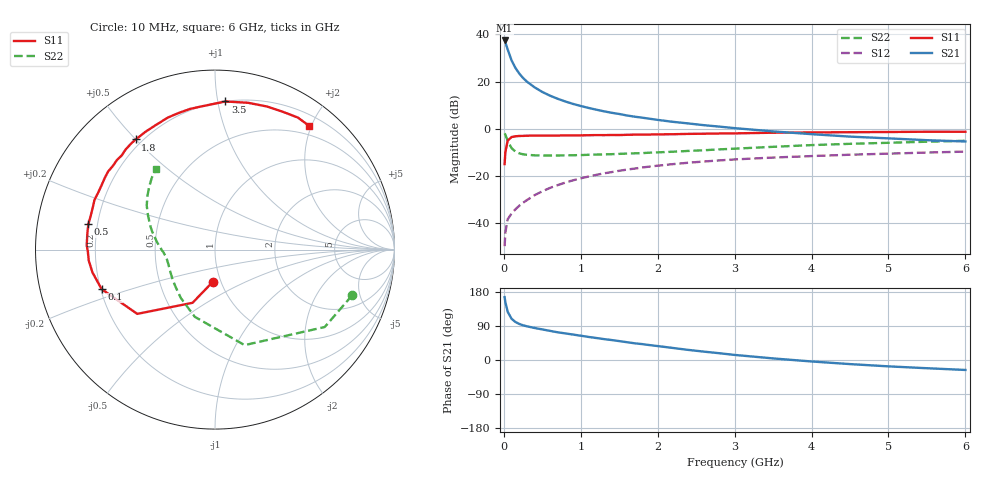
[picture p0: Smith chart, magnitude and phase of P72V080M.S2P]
! SIEMENS Small Signal Semiconductors
! BFP196
! Si NPN RF Bipolar Junction Transistor in SOT143
! VCE = 2 V  IC = 80 mA
! Common Emitter S-Parameters:  May  1996
# GHz  S  MA  R  50
!  f  S11  S21  S12  S22
! GHz  MAG  ANG  MAG  ANG  MAG  ANG  MAG  ANG
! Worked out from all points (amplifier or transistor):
!   36 points, 10 MHz to 6 GHz, reference 50 ohm
!   highest |S21| = 37.4 dB at 10 MHz (marker M1)
!   |S21| within 3 dB of that: start of sweep to 41.76 MHz
!   unconditionally stable (mu >= 1): 317.2 MHz to 5.129 GHz
!   at 250 MHz: K = 0.95, MSG = 26.4 dB, |S12| = -31.3 dB
!   at 1.4 GHz: K = 1.10, MAG = 10.6 dB, |S12| = -18.3 dB
!   at 6 GHz: K = 1.00, MSG = 2.1 dB, |S12| = -9.6 dB
!   S11 on the Smith chart (normalised r, x): 10 MHz: 0.92, -0.34; 100 MHz: 0.20, -0.16; 500 MHz: 0.16, +0.10; 1.8 GHz: 0.17, +0.50; 3.5 GHz: 0.20, +1.05; 6 GHz: 0.36, +1.97
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0.01  0.1794 -93.7  73.86 165.9  0.0033 74.0  0.8052 -18.5
0.02  0.3218 -112.9  67.38 152.5  0.0065 67.3  0.7483 -35.2
0.05  0.5619 -140.4  47.5 127.3  0.0122 55.1  0.5571 -72.8
0.1  0.6691 -160.8  28.14 108.9  0.0162 51.9  0.3911 -106.7
0.15  0.6946 -169.5  19.49 100.4  0.0198 53.8  0.3308 -124.9
0.2  0.7062 -175.1  14.82 95.2  0.0236 58.5  0.3031 -136.2
0.25  0.7083 -179.0  11.87 91.6  0.0273 60.4  0.2894 -144.4
0.3  0.7152 178.1  9.957 88.9  0.0311 62.8  0.2823 -149.5
0.4  0.7169 172.8  7.529 84.5  0.0396 64.9  0.2751 -157.2
0.5  0.7198 168.7  6.019 80.7  0.0477 66.0  0.2723 -162.0
0.6  0.7176 164.8  5.022 76.9  0.0563 66.2  0.2723 -165.3
0.7  0.7205 160.8  4.315 73.1  0.0645 65.9  0.273 -167.7
0.9  0.7241 154.2  3.364 67.1  0.0815 64.2  0.2762 -171.6
1.1  0.7323 147.1  2.767 60.9  0.098 62.1  0.2823 -174.5
1.4  0.7401 137.6  2.185 52.7  0.1215 57.6  0.2909 -178.0
1.8  0.7567 125.8  1.719 41.9  0.1521 51.6  0.3066 177.3
2.2  0.7686 115.2  1.404 31.7  0.1793 45.5  0.3279 172.1
2.8  0.7961 100.1  1.114 17.9  0.2146 36.3  0.3676 163.3
3.5  0.8273 86.0  0.882 4.2  0.2468 26.2  0.4163 153.5
4.5  0.8481 70.1  0.684 -10.8  0.2833 14.0  0.4815 141.4
5.5  0.8686 57.9  0.575 -21.7  0.3147 3.1  0.5338 131.2
6  0.8663 52.6  0.54 -26.3  0.3296 -2.6  0.5585 126.2
